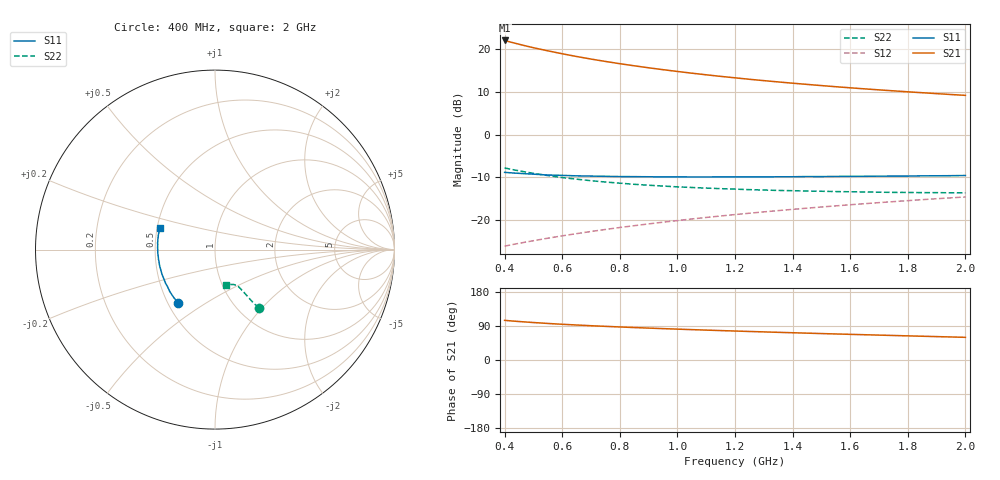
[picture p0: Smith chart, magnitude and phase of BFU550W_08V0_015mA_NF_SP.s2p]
! Filename:  P:\Prog\Test\Noise\ATS_data\Testdata_Net\06 Compressed Noise after Statistics\BFU550W_APM2013_11_D05_08p0V_015mA_NF_CM01_D.sf
! Date/Time: Tue 26/Mar/2013 16:25:26
! BFU550W_APM2013_11_D05_08p0V_1to35mA_NF_CM01_Bias7_R.sf
! Noise Parameter Data File
! BFU550W_APM2013_11_D05_08p0V_1to35mA_NF_CM01
! Date/time: Mon Mar 25 14:39:45 2013
! VAR V_out= 8.000000
! VAR I_out= 14.995000
! VAR V_in= 0.807400
! VAR I_in= 0.149500
! Device data file deembeded for feedlines and parallel
! Original file: \06 Compressed Noise after Statistics\BFU550W_APM2013_11_D05_08p0V_015mA_NF_CM01_R.sf
! Feed-files: PR019V01_070313_Feed1.s2p, PR019V01_070313_Feed2.s2p
! Parallel-file: PR019V01_070313_Par.s2p
# MHz S MA R 50
!  Freq-MHz  S11-mag  S11-arg  S21-mag  S21-arg  S12-mag  S12-arg  S22-mag  S22-arg
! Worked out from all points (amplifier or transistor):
!   37 points, 400 MHz to 2 GHz, reference 50 ohm
!   highest |S21| = 22.0 dB at 400 MHz (marker M1)
!   |S21| within 3 dB of that: start of sweep to 591.7 MHz
!   unconditionally stable (mu >= 1): 1.244 GHz to end of sweep
!   at 500 MHz: K = 0.83, MSG = 22.6 dB, |S12| = -24.8 dB
!   at 1.1 GHz: K = 0.99, MSG = 16.7 dB, |S12| = -19.4 dB
!   at 2 GHz: K = 1.01, MAG = 11.3 dB, |S12| = -14.6 dB
!   lowest NFmin = 0.83 dB at 400 MHz
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400  0.3609 -124.9  12.6 104.6  0.0494 62.4  0.4061 -53.0
420  0.3568 -127.6  12.08 103.3  0.05099 62.6  0.3938 -53.4
440  0.3532 -130.2  11.61 102.1  0.05256 62.8  0.3817 -53.7
460  0.3496 -132.5  11.16 101.0  0.0541 63.0  0.3709 -54.0
500  0.3437 -137.1  10.37 98.9  0.05722 63.5  0.3515 -54.5
550  0.3358 -141.8  9.531 96.4  0.06121 64.2  0.331 -55.0
600  0.3327 -146.3  8.806 94.3  0.06524 64.6  0.3136 -55.2
650  0.3284 -150.1  8.179 92.3  0.06925 65.1  0.3003 -55.6
700  0.3263 -153.8  7.636 90.5  0.07338 65.5  0.2882 -55.9
750  0.3243 -157.0  7.161 88.8  0.07747 65.9  0.278 -56.1
800  0.3222 -160.1  6.741 87.2  0.08166 66.2  0.2697 -56.6
850  0.3215 -163.0  6.369 85.6  0.08576 66.4  0.2615 -56.7
950  0.3192 -167.9  5.737 82.8  0.09425 66.8  0.2495 -57.4
1050  0.3188 -172.4  5.22 80.2  0.1028 67.0  0.2401 -58.3
1150  0.3196 -176.6  4.79 77.7  0.1114 67.1  0.2326 -59.2
1200  0.319 -178.3  4.605 76.5  0.1157 67.0  0.2296 -59.9
1250  0.3193 179.7  4.429 75.3  0.12 67.0  0.2265 -60.2
1350  0.3201 176.5  4.123 73.0  0.1288 66.8  0.2217 -61.5
1500  0.3218 171.7  3.737 69.8  0.1419 66.3  0.2169 -63.7
1650  0.3244 167.3  3.421 66.7  0.1552 65.8  0.2128 -65.9
1750  0.3263 164.8  3.243 64.7  0.164 65.3  0.2103 -67.6
2000  0.3316 158.4  2.872 59.8  0.1861 63.9  0.2075 -72.5
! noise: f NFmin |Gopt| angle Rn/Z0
400  0.8294  0.1797  178  0.0746
460  0.8512  0.1993  -179  0.0692
600  0.9015  0.1949  -178.7  0.0725
800  0.915  0.2114  -174.8  0.0712
1000  0.9306  0.2263  -173  0.0705
1200  0.9634  0.2492  -171.2  0.0686
1400  0.9811  0.2642  -165.7  0.0714
1600  1.022  0.2746  -164  0.0721
1800  1.028  0.2982  -157.4  0.0753
2000  1.069  0.3185  -157.1  0.0747
